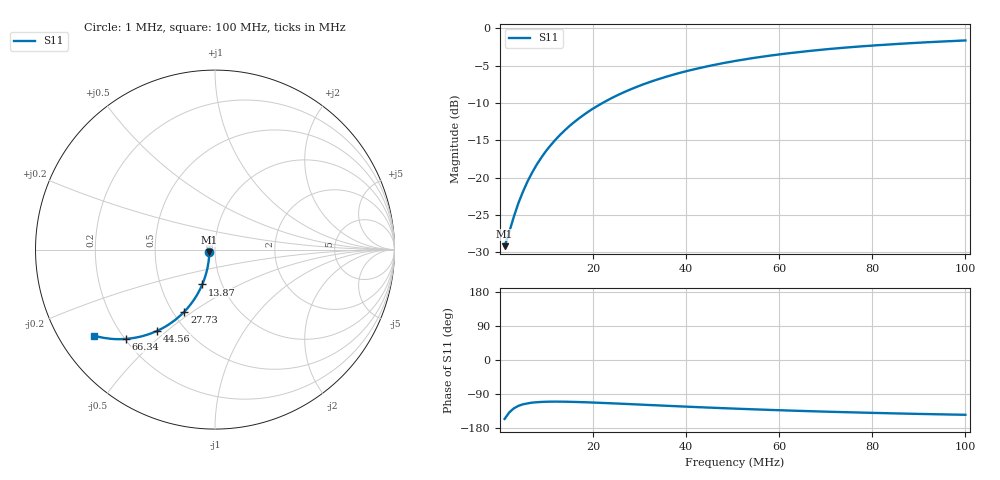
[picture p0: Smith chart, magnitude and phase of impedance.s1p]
# Hz S RI R 50.0
! written by SimSmith version 18.3b
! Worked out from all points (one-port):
!   101 points, 1 MHz to 100 MHz, reference 50 ohm
!   lowest |S11| = -29.2 dB at 1 MHz (marker M1), VSWR 1.07, Z = 46.9 - j1.35 ohm
!   |S11| at or under -10 dB: start of sweep to 22.08 MHz
!   S11 on the Smith chart (normalised r, x): 1 MHz: 0.94, -0.03; 13.87 MHz: 0.81, -0.33; 27.73 MHz: 0.57, -0.46; 44.56 MHz: 0.35, -0.46; 66.34 MHz: 0.20, -0.40; 100 MHz: 0.10, -0.32
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1000000  -0.0317 -0.0144
1990000  -0.0323 -0.0287
2980000  -0.0334 -0.0433
3970000  -0.0348 -0.058
4960000  -0.0365 -0.0721
5950000  -0.0392 -0.0861
6940000  -0.0413 -0.1003
7930000  -0.0447 -0.1141
8920000  -0.0482 -0.1278
9910000  -0.0521 -0.1417
1.189e7  -0.0606 -0.1682
1.387e7  -0.0708 -0.194
1.486e7  -0.0765 -0.2067
1.684e7  -0.0884 -0.2309
1.981e7  -0.1088 -0.2658
2.278e7  -0.1305 -0.2977
2.575e7  -0.154 -0.3276
2.773e7  -0.1709 -0.3457
3.268e7  -0.2147 -0.3857
3.862e7  -0.2687 -0.4241
4.456e7  -0.3221 -0.4525
5.05e7  -0.3741 -0.4732
5.644e7  -0.4229 -0.4866
6.337e7  -0.4757 -0.4952
6.634e7  -0.4971 -0.4972
7.525e7  -0.5543 -0.4987
8.812e7  -0.6235 -0.491
1e8  -0.6745 -0.4794
